//{{V2}}
ORGANIZATION_BLOCK OB100
TITLE= "Complete Restart"


AUTHOR:nb
FAMILY:nb
NAME:nb
VERSION:00.01


VAR_TEMP
       OB100_EV_CLASS:BYTE //16#13, Event class 1, Entering event state, Event logged in diagnostic buffer
       OB100_STRTUP:BYTE //16#81/82/83/84 Method of startup
       OB100_PRIORITY:BYTE //Priority of OB Execution
       OB100_OB_NUMBR:BYTE //100 (Organization block 100, OB100)
       OB100_RESERVED_1:BYTE //Reserved for system
       OB100_RESERVED_2:BYTE //Reserved for system
       OB100_STOP:WORD //Event that caused CPU to stop (16#4xxx)
       OB100_STRT_INFO:DWORD //Information on how system started
       OB100_DATE_TIME:DATE_AND_TIME //Date and time OB100 started
END_VAR
BEGIN

NETWORK
TITLE=
//{{a}}
//

       L    0
       T    MB        0

       T    MB      219

END_ORGANIZATION_BLOCK
